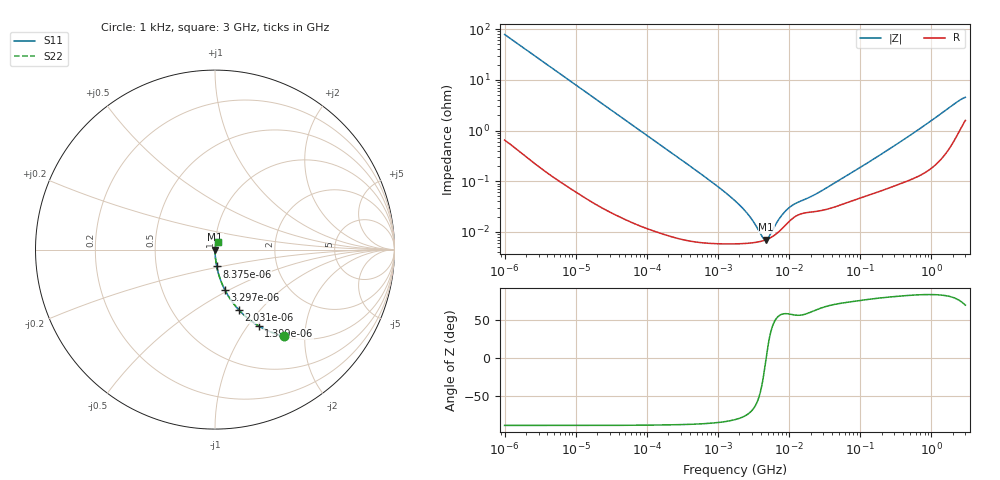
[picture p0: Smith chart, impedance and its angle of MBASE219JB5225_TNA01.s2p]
! MBASE219JB5225_TNA01  S-PARAMETER MODEL  ( Standard Model )
! Model Generated by TAIYO YUDEN Corporation (http://www.ty-top.com)
! Version 1.0
! TAIYO YUDEN Control No. 220601
! Copyright(c) 2012 TAIYO YUDEN CO.,LTD. All Rights Reserved.
! Product Description (link to TY-COMPAS)
! https://ds.yuden.co.jp/TYCOMPAS/or/detail?pn=MBASE219JB5225KTNA01&u=M
! Products Name : Multilayer Ceramic Capacitors
! Characteristics :
!  Capacitance : 2.2 [uF] , Rated Voltage : 16 [V] , TCC : X5R
!  Case Size : 2.0 x 1.25 / 0.079 x 0.049 [mm/inch] , Thickness : 0.85 / 0.033 [mm/inch]
!  (Conditions: Temperature = 25 [degC] , DC Bias Voltage = 0 [V])
! External Node Assignments :
!  1  o---| |---o  2
! GND o---------o GND
! Frequency Range : 1kHz  -  3GHz  [ 401 STEP ]
# MHZ S RI R 50
! Freq[MHz].  S11 Real  S11 Imag  S21 Real  S21 Imag  S12 Real  S12 Imag  S22 Real  S22 Imag
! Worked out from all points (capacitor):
!   401 points, 1 kHz to 3 GHz, reference 50 ohm
!   read as one part in series: C = 2.02 uF near 1.077 kHz
!   lowest |Z| = 7 mohm at 4.74 MHz (marker M1)
!   series resonance near 4.753 MHz, so ESL is about 550 pH
!   S11 on the Smith chart (normalised r, x): 1 kHz: 1.01, -1.57; 1.399 kHz: 1.01, -1.13; 2.031 kHz: 1.01, -0.78; 3.297 kHz: 1.00, -0.48; 8.375 kHz: 1.00, -0.19; 3 GHz: 1.03, +0.08
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0.001  0.3826 -0.4819  0.6174 0.4819  0.6174 0.4819  0.3826 -0.4819
0.001399  0.2424 -0.4245  0.7576 0.4245  0.7576 0.4245  0.2424 -0.4245
0.002031  0.133 -0.3358  0.867 0.3358  0.867 0.3358  0.133 -0.3358
0.003297  0.0558 -0.226  0.9442 0.226  0.9442 0.226  0.0558 -0.226
0.008375  0.0096 -0.0938  0.9904 0.0938  0.9904 0.0938  0.0096 -0.0938
0.01216  0.00476 -0.065  0.9952 0.065  0.9952 0.065  0.00476 -0.065
0.033275  0.000804 -0.024  0.9992 0.024  0.9992 0.024  0.000804 -0.024
0.147855  0.000125 -0.00544  0.9999 0.00544  0.9999 0.00544  0.000125 -0.00544
0.791611  6.01e-05 -0.000995  0.9999 0.000995  0.9999 0.000995  6.01e-05 -0.000995
1.732051  5.81e-05 -0.000407  0.9999 0.000407  0.9999 0.000407  5.81e-05 -0.000407
2.610246  5.95e-05 -0.000219  0.9999 0.000219  0.9999 0.000219  5.95e-05 -0.000219
3.789741  6.39e-05 -7.91e-05  0.9999 7.91e-05  0.9999 7.91e-05  6.39e-05 -7.91e-05
4.083148  6.55e-05 -5.29e-05  0.9999 5.29e-05  0.9999 5.29e-05  6.55e-05 -5.29e-05
4.739869  7e-05 -9.23e-07  0.9999 9.23e-07  0.9999 9.23e-07  7e-05 -9.23e-07
5.30084  7.5e-05 3.82e-05  0.9999 -3.82e-05  0.9999 -3.82e-05  7.5e-05 3.82e-05
5.711239  7.94e-05 6.45e-05  0.9999 -6.45e-05  0.9999 -6.45e-05  7.94e-05 6.45e-05
7.988506  0.000117 0.000184  0.9999 -0.000184  0.9999 -0.000184  0.000117 0.000184
10.37087  0.000168 0.000264  0.9998 -0.000264  0.9998 -0.000264  0.000168 0.000264
21.06097  0.000247 0.000447  0.9998 -0.000447  0.9998 -0.000447  0.000247 0.000447
256.0921  0.000756 0.00425  0.9992 -0.00425  0.9992 -0.00425  0.000756 0.00425
2310.849  0.00935 0.0353  0.9906 -0.0353  0.9906 -0.0353  0.00935 0.0353
3000  0.0173 0.041  0.9827 -0.041  0.9827 -0.041  0.0173 0.041
